(* IEC 60870-5-101 system configuration parameter *)
TYPE ST_IEC870_5_101MSysPara :
STRUCT
	asduAddr	: WORD := 1;(* Common address of ASDU *)
	nOrg		: BYTE := 0;(* Originator address *)

	asduFmt		: ST_IEC870_5_101AsduFmtParams := ( eCOTSize := eIEC870_COT_OneOctet,
													eAsduAddrSize := eIEC870_AsduAddr_OneOctet,
													eObjAddrSize := eIEC870_ObjAddr_TwoOctets );(* ASDU frame format parameter (octet lengths) *)

	bTest		: BOOL := FALSE;(* Enable/disable cyclic test command *)
	tTest		: TIME := T#10S;(* Test command cycle time *)

	bClock		: BOOL := FALSE;(* Enable/disable cyclic clock synchronisation command *)
	tClock		: TIME := T#20s;(* Clock synchronisation cycle time *)

	bGenin		: BOOL := FALSE;(* Enable/disable cyclic general interrogation command *)
	eGeninQoi	: E_IEC870_5_101QOI := eIEC870_QOI_INROGEN;(* Qualifier of general interrogation command *)
	tGenin		: TIME := T#40S;(* General interrogation cycle time *)

	bCoro		: BOOL := FALSE;(* Enable/disable general counter interrogation command *)
	eCoroMode	: E_IEC870_5_101CoroMode := eIEC870_CoroMode_A;(* Counter interrogation operation mode *)
	bCoroReset	: BOOL := FALSE;(* FALSE => Freeze counter values, TRUE => Freeze and reset counter values *)
	eCoroRqt	: E_IEC870_5_101RQT := eIEC870_RQT_REQCOGEN;(* Request qualifier of counter interrogation command *)
	tCoro		: TIME := T#60S;(* Counter interrogation cycle time *)

	tCon		: TIME := T#5S;(* Max. command activation confirmation timeout time *)
	tTerm		: TIME := T#60S;(* Max. command activation termination timeout time *)

	bDbgLink 	: BOOL := FALSE;(* TRUE => Log serial link layer frames to TwinCAT output window *)
	bDbgAppl	: BOOL := FALSE;(* TRUE => Log application layer messages immediatelly to TwinCAT output window *)
	eDbgAsdu 	: E_IEC870_5_101FifoDbgFlags := eIEC870_FIFO_DBG_OFF;(* eIEC870_FIFO_DBG_ALL => Log ASDU TX/RX fifo frames to TwinCAT output window *)
END_STRUCT
END_TYPE
